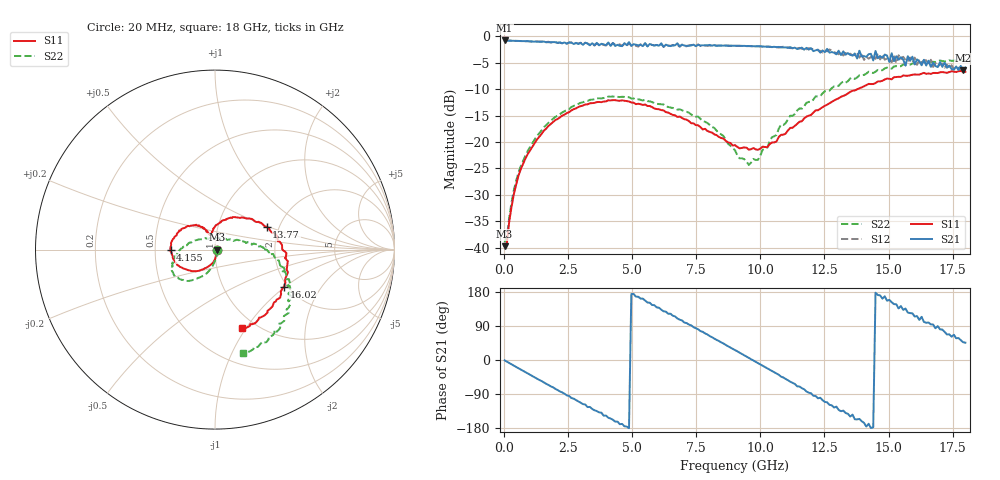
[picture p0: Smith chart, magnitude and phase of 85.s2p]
!Agilent Technologies,N5230A,US43500223,A.07.50.48
!Agilent N5230A: A.07.50.48
!Date: Saturday, January 16, 2016 20:59:30
!Correction: S11(Full 2 Port(1,2))
!S21(Full 2 Port(1,2))
!S12(Full 2 Port(1,2))
!S22(Full 2 Port(1,2))
!S2P File: Measurements: S11, S21, S12, S22:
# Hz S  dB  R 50
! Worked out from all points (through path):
!   201 points, 20 MHz to 18 GHz, reference 50 ohm
!   highest |S21| = -0.78 dB at 20 MHz (marker M1); lowest = -6.4 dB at 17.91 GHz (marker M2)
!   group delay of S21, straight-line fit = 104 ps
!   lowest |S11| = -39.7 dB at 20 MHz (marker M3), VSWR 1.02, Z = 51 - j0.124 ohm
!   |S11| at or under -10 dB: start of sweep to 13.79 GHz
!   |S22| runs from -39.0 to -4.4 dB; largest |S21 - S12| = 0.14
!   S11 on the Smith chart (normalised r, x): 20 MHz: 1.02, -0.00; 4.155 GHz: 0.60, -0.00; 13.77 GHz: 1.72, +0.49; 16.02 GHz: 1.92, -0.98; 18 GHz: 0.86, -0.96
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2e7  -39.70 -6.7  -0.78 -0.9  -0.79 -0.8  -38.97 -5.6
4.695e8  -28.07 -83.7  -0.86 -18.3  -0.86 -18.3  -27.34 -79.8
9.19e8  -22.31 -100.2  -0.90 -35.4  -0.92 -35.4  -21.70 -96.2
1.9978e9  -15.85 -131.6  -1.11 -76.1  -1.13 -76.8  -15.26 -117.7
3.0766e9  -13.10 -156.3  -1.60 -116.4  -1.50 -115.8  -12.47 -133.1
4.1554e9  -12.13 -179.2  -1.80 -154.5  -1.74 -154.2  -11.42 -147.5
4.8746e9  -12.33 166.3  -1.09 -179.9  -1.31 179.9  -11.52 -156.4
6.0433e9  -13.79 141.7  -1.76 138.0  -1.92 138.3  -12.81 -169.4
7.5716e9  -16.83 118.6  -1.60 81.0  -1.53 80.7  -15.19 172.6
9.01e9  -20.58 111.0  -1.78 26.2  -1.81 26.6  -21.54 130.5
9.5494e9  -21.46 107.2  -1.83 5.6  -1.85 6.0  -24.33 92.0
1.03585e10  -20.44 101.3  -1.94 -25.5  -2.00 -25.3  -19.87 34.5
1.11676e10  -17.32 88.1  -2.04 -57.4  -2.23 -57.4  -15.02 12.8
1.20666e10  -14.42 66.5  -2.80 -94.4  -2.43 -91.4  -11.97 4.5
1.30555e10  -11.72 41.9  -2.72 -131.8  -3.40 -130.7  -9.37 -9.2
1.37747e10  -10.03 23.9  -4.19 -156.7  -3.14 -159.6  -7.79 -17.3
1.44939e10  -8.84 7.5  -2.77 177.6  -4.24 -178.6  -6.69 -25.8
1.50333e10  -8.04 -6.5  -4.84 158.6  -4.39 154.0  -6.05 -35.1
1.60222e10  -7.21 -28.2  -5.32 114.8  -4.03 120.9  -5.18 -48.4
1.70111e10  -6.80 -50.1  -4.87 80.7  -5.35 85.8  -4.58 -61.0
1.79101e10  -6.68 -70.5  -6.42 46.9  -5.99 48.7  -4.55 -73.8
1.8e10  -6.72 -71.1  -5.92 45.7  -6.50 46.5  -4.50 -74.8
